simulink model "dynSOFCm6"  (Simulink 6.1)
settings: Solver=ode15s  StartTime=0.0  StopTime=1000  FixedStep=0.001  MinStep=1e-10  RelTol=1e-3
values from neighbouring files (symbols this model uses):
  A = 1e-4    (= 0.0001)    [dynSOFC_par.m]
  Aa = r3^2*(4-pi)    (= 0.000103867288916)    [dynSOFC_par.m]
  Ac = pi*(r2^2-r1^2)    (= 0.000122508290482)    [dynSOFC_par.m]
  At = pi*r0^2    (= 7.85398163397e-05)    [dynSOFC_par.m]
  C = 300e-6    (= 0.0003)    [dynSOFC_par.m]
  Cpc = 740    [dynSOFC_par.m]
  Cpt = 1217.7    [dynSOFC_par.m]
  D_a = 0.273*2*r3    (= 0.006006)    [dynSOFC_par.m]
  D_c = 2*(r2-r1)    (= 0.00532)    [dynSOFC_par.m]
  delta = 5.67e-8    (= 5.67e-08)    [dynSOFC_par.m]
  dVa = Aa*A/(2*pi*r3)    (= 1.50281749604e-07)    [dynSOFC_par.m]
  dVc = Ac*A/(2*pi*r3)    (= 1.77252727273e-07)    [dynSOFC_par.m]
  dVt = At*A/(2*pi*r3)    (= 1.13636363636e-07)    [dynSOFC_par.m]
  Ea = 1.1e5    (= 110000)    [dynSOFC_par.m]
  Ec = 1.2e5    (= 120000)    [dynSOFC_par.m]
  Ems1 = 0.4    [dynSOFC_par.m]
  Ems2 = 0.9    [dynSOFC_par.m]
  F = 96487    [dynSOFC_par.m]
  F21 = 0.69    [dynSOFC_par.m]
  K = 10    [dynSOFC_par.m]
  La = 0.1e-3    (= 0.0001)    [dynSOFC_par.m]
  Lc = 2.21e-3    (= 0.00221)    [dynSOFC_par.m]
  Le = 0.04e-3    (= 4e-05)    [dynSOFC_par.m]
  R = 8.314/101325    (= 8.20528003948e-05)    [dynSOFC_par.m]
  r0 = 5e-3    (= 0.005)    [dynSOFC_par.m]
  r1 = 6e-3    (= 0.006)    [dynSOFC_par.m]
  r2 = 8.66e-3    (= 0.00866)    [dynSOFC_par.m]
  r3 = 11e-3    (= 0.011)    [dynSOFC_par.m]
  Ro = 0.01    [dynSOFC_par.m]
  Rouc = 4592    [dynSOFC_par.m]
  Rout = 3900    [dynSOFC_par.m]
  x_ini = [    [dynSOFC_par.m]
libraries: simulink x25
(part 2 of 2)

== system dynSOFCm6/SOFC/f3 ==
  note: 1-4
  note: 5-6
  note: 7-10
  note: 11
  note: x1-3
  note: u1
  note: x17,22
  x : Inport  Port=1  LatchInput=off
  u : Inport  Port=2  LatchInput=off
  DH2 : Inport  Port=3  LatchInput=off
  Derivative1 : Derivative
  Ex3 : Fcn  Expr=-u(7)*u(2) - u(8)*u(3) + u(7)/(2*F)*(u(1)/u(5)) + u(9)*A/R/u(11)*u(4)
  JsH2 : Selector  Elements=[1 2 3]  InputPortWidth=28
  Mux : Mux
  Mux1 : Mux
  Mux2 : Mux  Inputs=2
  Mux3 : Mux  Inputs=2
  Rload+Ro : Selector  Elements=[1]  InputPortWidth=16
  Tcell : Selector  Elements=[15]  InputPortWidth=28
  "Tfuel, NH2" : Selector  Elements=[17 22 ]  InputPortWidth=28
  Transfer Fcn : TransferFcn  Denominator=[0.001 1]
  a1 : Fcn  Expr=24*u(1)^2/(La^4)
  a2 : Fcn  Expr=12*u(1)/(La^2)
  a3 : Fcn  Expr=24*u(1)^2/(La^3)
  a4 : Fcn  Expr=24*u(1)/(La^3)
  pbH2 : Fcn  Expr=u(2)*u(1)*R/dVa
  dot x3 : Outport
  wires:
  x/1 -> JsH2/1, Tcell/1, "Tfuel, NH2"/1
  DH2/1 -> a1/1, a2/1, a4/1, a3/1
  a1/1 -> Mux/1
  a2/1 -> Mux/2
  a3/1 -> Mux/3
  a4/1 -> Mux/4
  Mux/1 -> Mux1/3
  Mux1/1 -> Ex3/1
  Ex3/1 -> dot x3/1
  Tcell/1 -> Mux1/4
  "Tfuel, NH2"/1 -> pbH2/1
  Mux2/1 -> Mux1/2
  Rload+Ro/1 -> Mux2/1
  pbH2/1 -> Mux2/2, Derivative1/1
  u/1 -> Rload+Ro/1
  JsH2/1 -> Mux3/1
  Mux3/1 -> Mux1/1
  Derivative1/1 -> Transfer Fcn/1
  Transfer Fcn/1 -> Mux3/2

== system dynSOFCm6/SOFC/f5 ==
  note: 7-10
  note: 5-6
  note: 1-4
  note: 11
  note: x18,24
  note: u1
  note: x1,4,5
  note: x15
  x : Inport  Port=1  LatchInput=off
  u : Inport  Port=2  LatchInput=off
  DO2 : Inport  Port=3  LatchInput=off
  Derivative1 : Derivative
  Ex5 : Fcn  Expr=-u(7)*u(2) - u(8)*u(3) + u(7)/(4*F)*(u(1)/u(5)) + u(9)*A/R/u(11)*u(4)
  JsO2 : Selector  Elements=[1 4 5]  InputPortWidth=28
  Mux : Mux
  Mux1 : Mux
  Mux2 : Mux  Inputs=2
  Mux3 : Mux  Inputs=2
  Rload+Ro : Selector  Elements=[1]  InputPortWidth=16
  "Tair, NO2" : Selector  Elements=[18 24 ]  InputPortWidth=28
  Tcell : Selector  Elements=[15]  InputPortWidth=28
  Transfer Fcn : TransferFcn  Denominator=[0.001 1]
  a1 : Fcn  Expr=24*u(1)^2/(Lc^4)
  a2 : Fcn  Expr=12*u(1)/(Lc^2)
  a3 : Fcn  Expr=24*u(1)^2/(Lc^3)
  a4 : Fcn  Expr=24*u(1)/(Lc^3)
  pbO2 : Fcn  Expr=u(2)*u(1)*R/dVc
  dot x5 : Outport
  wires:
  Ex5/1 -> dot x5/1
  Mux1/1 -> Ex5/1
  Mux/1 -> Mux1/3
  a4/1 -> Mux/4
  a3/1 -> Mux/3
  a2/1 -> Mux/2
  a1/1 -> Mux/1
  DO2/1 -> a3/1, a4/1, a2/1, a1/1
  x/1 -> JsO2/1, Tcell/1, "Tair, NO2"/1
  u/1 -> Rload+Ro/1
  Tcell/1 -> Mux1/4
  "Tair, NO2"/1 -> pbO2/1
  Rload+Ro/1 -> Mux2/1
  pbO2/1 -> Mux2/2, Derivative1/1
  Mux2/1 -> Mux1/2
  JsO2/1 -> Mux3/1
  Mux3/1 -> Mux1/1
  Derivative1/1 -> Transfer Fcn/1
  Transfer Fcn/1 -> Mux3/2

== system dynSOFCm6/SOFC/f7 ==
  note: 1-4
  note: 5-6
  note: 7-10
  note: 11
  note: u1
  note: x20,24
  note: x1,6,7
  note: x15
  x : Inport  Port=1  LatchInput=off
  u : Inport  Port=2  LatchInput=off
  DH2O : Inport  Port=3  LatchInput=off
  Derivative1 : Derivative
  Ex9 : Fcn  Expr=-u(7)*u(2) - u(8)*u(3) + u(7)/(2*F)*(-u(1)/u(5)) + u(9)*A/R/u(11)*u(4)
  JsH2O : Selector  Elements=[1 6 7]  InputPortWidth=28
  Mux : Mux
  Mux1 : Mux
  Mux2 : Mux  Inputs=2
  Mux3 : Mux  Inputs=2
  Rload+Ro : Selector  Elements=[1]  InputPortWidth=16
  Tcell : Selector  Elements=[15]  InputPortWidth=28
  "Tfuel, NH2O" : Selector  Elements=[17 21 ]  InputPortWidth=28
  Transfer Fcn : TransferFcn  Denominator=[0.001 1]
  a1 : Fcn  Expr=24*u(1)^2/(Lc^4)
  a2 : Fcn  Expr=12*u(1)/(Lc^2)
  a3 : Fcn  Expr=24*u(1)^2/(Lc^3)
  a4 : Fcn  Expr=24*u(1)/(Lc^3)
  pbH2O : Fcn  Expr=u(2)*u(1)*R/dVa
  dot x7 : Outport
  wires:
  u/1 -> Rload+Ro/1
  x/1 -> JsH2O/1, Tcell/1, "Tfuel, NH2O"/1
  DH2O/1 -> a1/1, a2/1, a4/1, a3/1
  a1/1 -> Mux/1
  a2/1 -> Mux/2
  a3/1 -> Mux/3
  a4/1 -> Mux/4
  Mux/1 -> Mux1/3
  Mux1/1 -> Ex9/1
  Ex9/1 -> dot x7/1
  Tcell/1 -> Mux1/4
  "Tfuel, NH2O"/1 -> pbH2O/1
  Rload+Ro/1 -> Mux2/1
  pbH2O/1 -> Mux2/2, Derivative1/1
  Mux2/1 -> Mux1/2
  JsH2O/1 -> Mux3/1
  Mux3/1 -> Mux1/1
  Derivative1/1 -> Transfer Fcn/1
  Transfer Fcn/1 -> Mux3/2

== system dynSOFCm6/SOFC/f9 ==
  note: 7-10
  note: 5-6
  note: 1-4
  note: 11
  note: 12
  note: u1
  note: x20,25
  note: x1,8,9,14
  note: x15
  x : Inport  Port=1  LatchInput=off
  u : Inport  Port=2  LatchInput=off
  DH2 : Inport  Port=3  LatchInput=off
  dotx1 : Inport  Port=4  LatchInput=off
  Ex9 : Fcn  Expr=-u(7)*u(2) - u(8)*u(3) - R*u(12)/A/(2*F)*u(10)*u(1)/u(5) + u(7)*u(6) - R*u(12)/A*4/La/(2*F)*(u(11)/u(5) - u(1)/(u(5)^2)*(K*u(5)-u(4)))
  Mux : Mux
  Mux1 : Mux  Inputs=5
  Mux2 : Mux  Inputs=2
  Rload+Ro : Selector  Elements=[1]  InputPortWidth=16
  Tcell : Selector  Elements=[15]  InputPortWidth=28
  "Tfuel, NH2" : Selector  Elements=[17 22 ]  InputPortWidth=28
  a1 : Fcn  Expr=24*u(1)^2/(La^4)
  a2 : Fcn  Expr=12*u(1)/(La^2)
  a3 : Fcn  Expr=24*u(1)^2/(La^3)
  a4 : Fcn  Expr=24*u(1)/(La^3)
  pbH2 : Fcn  Expr=u(2)*u(1)*R/dVa
  ptH2 : Selector  Elements=[1 8 9 14]  InputPortWidth=28
  dot x9 : Outport
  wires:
  Ex9/1 -> dot x9/1
  Mux1/1 -> Ex9/1
  Mux/1 -> Mux1/3
  ptH2/1 -> Mux1/1
  a4/1 -> Mux/4
  a3/1 -> Mux/3
  a2/1 -> Mux/2
  a1/1 -> Mux/1
  DH2/1 -> a3/1, a4/1, a2/1, a1/1
  x/1 -> ptH2/1, Tcell/1, "Tfuel, NH2"/1
  dotx1/1 -> Mux1/4
  Tcell/1 -> Mux1/5
  "Tfuel, NH2"/1 -> pbH2/1
  Mux2/1 -> Mux1/2
  Rload+Ro/1 -> Mux2/1
  pbH2/1 -> Mux2/2
  u/1 -> Rload+Ro/1

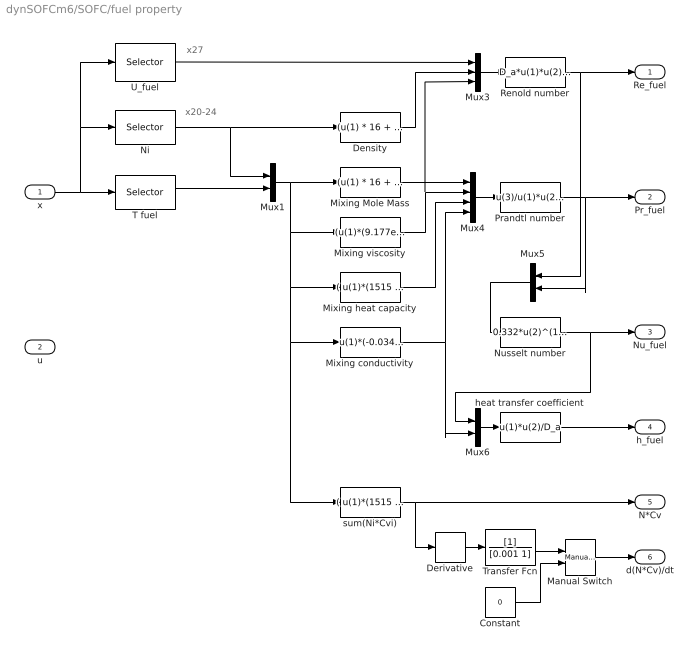
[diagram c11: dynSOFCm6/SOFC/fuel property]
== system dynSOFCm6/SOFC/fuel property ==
  note: x20-24
  note: x27
  x : Inport  Port=1  LatchInput=off
  u : Inport  Port=2  LatchInput=off
  Constant : Constant  Value=0
  Density : Fcn  Expr=(u(1) * 16 + u(2) * 18 + u(3) * 2 + u(4) *28 + u(5) *44) /dVa/1000
  Derivative : Derivative
  Manual Switch : simulink/Signal Routing/Manual Switch  sw=1  action=0
  Mixing Mole Mass : Fcn  Expr=(u(1) * 16 + u(2) * 18 + u(3) * 2 + u(4) *28 + u(5) *44) / (u(1) + u(2) + u(3) + u(4) + u(5))
  Mixing conductivity : Fcn  Expr="u(1)*(-0.03442 + 1.987e-4*u(6)) + u(2)*(-0.01450 + 9.782e-5*u(6)) + u(3)*(0.08525 + 2.964e-4*u(6)) + u(4)*(0.01275 + 5.348e-5*u(6)) + u(5)*(0.005485 + 6.272e-5*u(6))  / (u(1) + u(2) + u(3) + u(4) + u(5))"
  Mixing heat capacity : Fcn  Expr="( u(1)*(1515 + 83.47*u(6) -0.02053*u(6)^2)  + u(2)*(2.075e4 + 12.15*u(6)) +  u(3)*(1.829e4 +3.719*u(6)) + u(4)*(1.966e4 + 5.019*u(6)) + u(5)*(2.369e4 + 31.01*u(6) - 0.008875*u(6)^2) )   /  (u(1) +u(2) + u(3) + u(4) +u(5) )"
  Mixing viscosity : Fcn  Expr="(u(1)*(9.177e-6 + 1.755e-8*u(6)) +  u(2)*(4.567e-6 + 2.209e-8*u(6)) + u(3)*(6.162e-6 + 1.145e-8*u(6)) + u(4)*(1.399e-5 + 2.582e-8*u(6)) + u(5)*(1.273e-5 + 2.822e-8*u(6)) ) / (u(1) +u(2) + u(3) + u(4) +u(5) )"
  Mux1 : Mux  Inputs=2
  Mux3 : Mux  Inputs=3
  Mux4 : Mux
  Mux5 : Mux  Orientation=left  Inputs=2
  Mux6 : Mux  Inputs=2
  Ni : Selector  Elements=[20 21 22 23 24]  InputPortWidth=28
  Nusselt number : Fcn  Expr=0.332*u(2)^(1/3)*u(1)^(1/2)
  Prandtl number : Fcn  Expr=u(3)/u(1)*u(2)/u(4)
  Renold number : Fcn  Expr=D_a*u(1)*u(2)/u(3)
  T fuel : Selector  Elements=[17]  InputPortWidth=28
  Transfer Fcn : TransferFcn  Denominator=[0.001 1]
  U_fuel : Selector  Elements=[27]  InputPortWidth=28
  heat transfer coefficient : Fcn  Expr=u(1)*u(2)/D_a
  sum(Ni*Cvi) : Fcn  Expr="( u(1)*(1515 + 83.47*u(6) -0.02053*u(6)^2)  + u(2)*(2.075e4 + 12.15*u(6)) +  u(3)*(1.829e4 +3.719*u(6)) + u(4)*(1.966e4 + 5.019*u(6)) + u(5)*(2.369e4 + 31.01*u(6) - 0.008875*u(6)^2) )   /  1000"
  Re_fuel : Outport
  Pr_fuel : Outport  Port=2
  Nu_fuel : Outport  Port=3
  h_fuel : Outport  Port=4
  N*Cv : Outport  Port=5
  d(N*Cv)/dt : Outport  Port=6
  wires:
  heat transfer coefficient/1 -> h_fuel/1
  Mux6/1 -> heat transfer coefficient/1
  Nusselt number/1 -> Mux6/1, Nu_fuel/1
  Mux5/1 -> Nusselt number/1
  Prandtl number/1 -> Mux5/2, Pr_fuel/1
  Mixing conductivity/1 -> Mux6/2, Mux4/4
  Mixing heat capacity/1 -> Mux4/3
  Mux4/1 -> Prandtl number/1
  Mixing viscosity/1 -> Mux4/2, Mux3/3
  Mixing Mole Mass/1 -> Mux4/1
  Renold number/1 -> Mux5/1, Re_fuel/1
  Mux3/1 -> Renold number/1
  Density/1 -> Mux3/2
  U_fuel/1 -> Mux3/1
  T fuel/1 -> Mux1/2
  x/1 -> T fuel/1, U_fuel/1, Ni/1
  Ni/1 -> Density/1, Mux1/1
  Mux1/1 -> Mixing Mole Mass/1, Mixing viscosity/1, Mixing heat capacity/1, Mixing conductivity/1, sum(Ni*Cvi)/1
  sum(Ni*Cvi)/1 -> N*Cv/1, Derivative/1
  Constant/1 -> Manual Switch/2
  Manual Switch/1 -> d(N*Cv)/dt/1
  Derivative/1 -> Transfer Fcn/1
  Transfer Fcn/1 -> Manual Switch/1

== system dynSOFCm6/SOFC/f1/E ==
  x : Inport  Port=1  LatchInput=off
  u : Inport  Port=2  LatchInput=off
  E0 : Fcn  Expr=1.2723-2.7645e-4*u(15)
  Eta_C : Fcn  Expr=8.314*u(15)/2/F*log(u(8)*(u(10)^0.5)/u(12))
  Eta_a : Fcn  Expr="2*8.314*u(4)/F/2 * (  log(u(3)/u(1)/2 +  (1+(u(3)/u(1)/2) ^2)^0.5  ) + log(u(3)/u(2)/2 +  (1+(u(3)/u(2)/2) ^2)^0.5 )/2   )"
  Eta_act : Display
  I : Fcn  Expr=u(1)/u(2)
  Iao : Display
  Ico : Display
  Mux : Mux
  Mux1 : Mux  Inputs=2
  Rload : Selector  Elements=[1]  InputPortWidth=16
  Sum : Sum  Inputs=++-
  Tcell : Selector  Elements=[15]  InputPortWidth=28
  Vct : Selector  Elements=[1]  InputPortWidth=28
  ia0 : Fcn  Expr=7e9 * u(8) * u(12) * exp(-Ea/8.314/u(15)) * A
  ic0 : Fcn  Expr=7e9 * (u(10)^0.25) * exp(-Ec/8.314/u(15) ) * A
  E : Outport
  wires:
  Tcell/1 -> Mux/4
  Sum/1 -> E/1
  Eta_a/1 -> Sum/3, Eta_act/1
  Eta_C/1 -> Sum/2
  E0/1 -> Sum/1
  Rload/1 -> Mux1/2
  Vct/1 -> Mux1/1
  Mux1/1 -> I/1
  u/1 -> Rload/1
  Mux/1 -> Eta_a/1
  I/1 -> Mux/3
  ia0/1 -> Iao/1, Mux/1
  ic0/1 -> Mux/2, Ico/1
  x/1 -> Tcell/1, Vct/1, ic0/1, ia0/1, Eta_C/1, E0/1
